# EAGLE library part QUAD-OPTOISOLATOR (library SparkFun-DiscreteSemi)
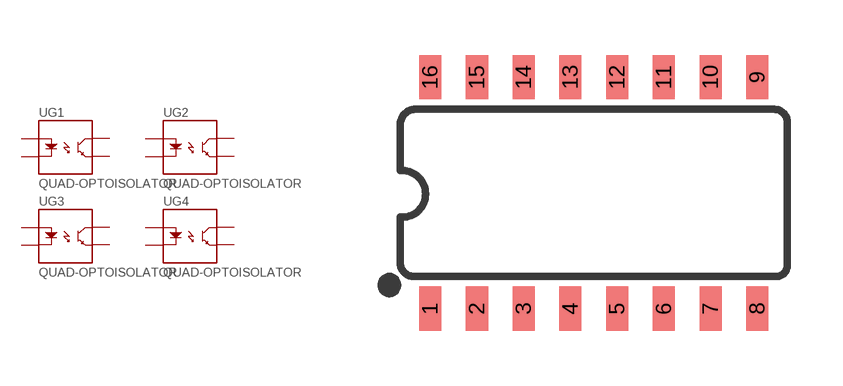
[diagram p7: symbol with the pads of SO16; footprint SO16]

Designator prefix U; gates G1=OPTOISOLATOR_SINGLE G2=OPTOISOLATOR_SINGLE G3=OPTOISOLATOR_SINGLE G4=OPTOISOLATOR_SINGLE

## QUAD-OPTOISOLATOR (PROD_ID: IC-14121; VALUE: TLP290-4)  [SO16]
1  G1:A1
2  G1:C1
3  G2:A1
4  G2:C1
5  G3:A1
6  G3:C1
7  G4:A1
8  G4:C1
9  G4:EM1
10  G4:CL1
11  G3:EM1
12  G3:CL1
13  G2:EM1
14  G2:CL1
15  G1:EM1
16  G1:CL1

## Footprint SO16 (pad centres in mm)
smd 0.6 x 1.2: 1 -4.445,-3.15; 2 -3.175,-3.15; 3 -1.905,-3.15; 4 -0.635,-3.15; 5 0.635,-3.15; 6 1.905,-3.15; 7 3.175,-3.15; 8 4.445,-3.15; 9 4.445,3.15; 10 3.175,3.15; 11 1.905,3.15; 12 0.635,3.15; 13 -0.635,3.15; 14 -1.905,3.15; 15 -3.175,3.15; 16 -4.445,3.15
